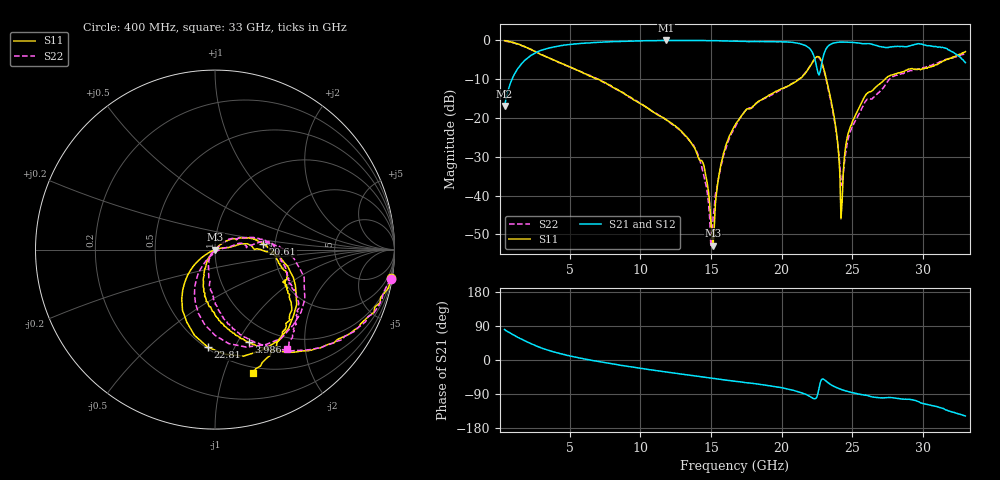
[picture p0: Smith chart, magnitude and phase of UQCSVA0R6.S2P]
!  Part Number  UQCSVA0R6  Mounting Orientation: Horizontal
!  Description: Ultra Low ESR Microwave capacitors
!  Application: Coupling, Bypass, Tuning, DC Block
!  Filters, Matching
# GHZ S DB R 50
! Freq  |S11|  S11 Ph  |S21|  S21 Ph  |S12|  S12 Ph  |S22|  S22 Ph
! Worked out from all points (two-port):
!   401 points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, 400 MHz to 33 GHz, reference 50 ohm
!   highest |S21| = 0.00 dB at 11.81 GHz (marker M1); lowest = -16.9 dB at 400 MHz (marker M2)
!   |S21| within 3 dB of the highest: 2.682 GHz to 22.16 GHz (19.48 GHz wide, 157 % of centre); 23.04 GHz to 32.12 GHz (9.082 GHz wide, 32.9 % of centre)
!   lowest |S11| = -52.9 dB at 15.15 GHz (marker M3), VSWR 1.00, Z = 50.2 - j0.0719 ohm
!   |S11| at or under -10 dB: 7.002 GHz to 21.24 GHz (14.24 GHz wide, 101 % of centre); 23.17 GHz to 27.31 GHz (4.143 GHz wide, 16.4 % of centre)
!   |S22| runs from -53.0 to 0.0 dB; largest |S21 - S12| = 0.014
!   S11 on the Smith chart (normalised r, x): 400 MHz: 1, -12; 3.986 GHz: 0.75, -1.11; 20.61 GHz: 1.72, +0.12; 22.81 GHz: 0.51, -0.79; 33 GHz: 0.44, -1.25
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0.4  -0.06 -9.2  -16.89 80.3  -16.84 80.1  -0.04 -9.6
1.623  -1.31 -34.7  -5.89 54.6  -5.91 53.6  -1.36 -36.5
3.986  -5.21 -70.1  -1.61 20.4  -1.63 20.3  -5.26 -68.2
5.861  -8.19 -87.1  -0.75 4.2  -0.74 4.3  -8.15 -82.5
11.321  -19.36 -118.7  -0.03 -28.9  -0.03 -28.9  -19.28 -109.2
11.81  -20.34 -120.5  0.00 -31.5  0.00 -31.3  -20.42 -112.8
14.418  -31.42 -122.8  -0.03 -45.0  -0.02 -44.9  -33.75 -131.2
14.907  -42.03 -119.3  -0.06 -47.3  -0.06 -47.2  -45.78 -111.4
15.152  -52.87 -18.4  -0.05 -48.5  -0.05 -48.3  -45.49 20.3
15.722  -31.62 44.4  -0.10 -51.5  -0.08 -51.3  -32.15 41.4
16.7  -21.90 36.9  -0.19 -56.0  -0.17 -56.2  -22.37 38.2
20.612  -11.43 6.8  -0.45 -78.3  -0.48 -78.3  -11.40 12.3
22.161  -5.79 -28.3  -3.00 -99.7  -2.98 -99.6  -5.68 -17.2
22.813  -5.28 -94.3  -6.34 -52.2  -6.34 -52.4  -5.52 -81.6
23.709  -19.55 -146.9  -0.64 -69.9  -0.68 -69.9  -20.25 -128.2
24.117  -34.28 -155.7  -0.42 -76.5  -0.47 -76.4  -32.06 -112.4
24.28  -41.47 12.7  -0.41 -78.7  -0.44 -78.6  -37.40 -45.9
24.606  -25.55 11.2  -0.44 -82.2  -0.49 -82.2  -27.18 8.5
25.013  -20.90 9.2  -0.49 -86.3  -0.55 -86.2  -22.17 10.3
27.621  -9.18 -8.6  -1.74 -99.1  -1.79 -98.8  -10.01 5.6
29.74  -7.40 -24.1  -0.85 -110.9  -0.87 -111.1  -7.39 -21.2
33  -2.88 -73.0  -5.73 -147.7  -5.75 -147.2  -3.30 -54.3
